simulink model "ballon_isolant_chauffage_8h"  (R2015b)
settings: Solver=ode23t  StartTime=0.0  StopTime=86400  RelTol=1e-3
undefined symbols (not defined in the file): sigbuilder_block
libraries: fl_lib x7, nesl_utility x4

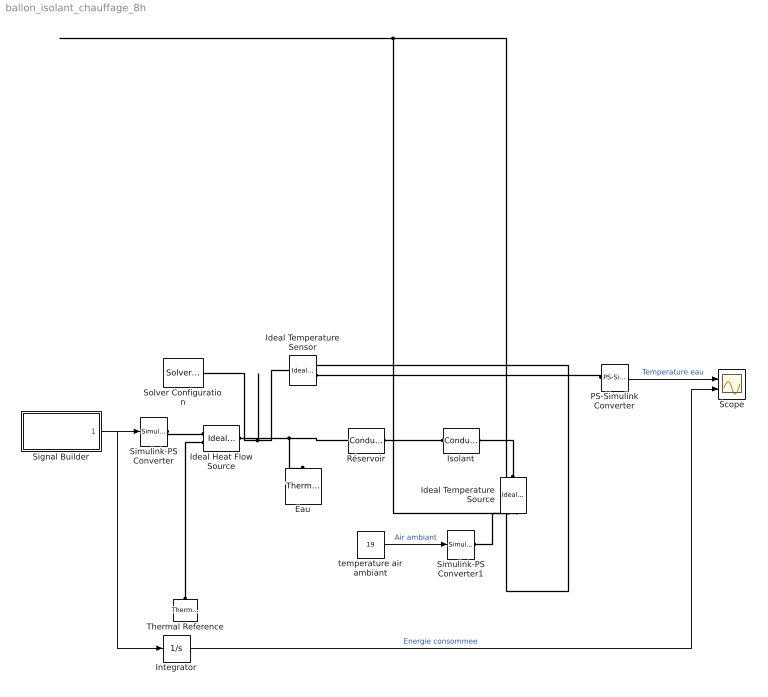
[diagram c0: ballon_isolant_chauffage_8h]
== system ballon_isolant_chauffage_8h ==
  Eau : fl_lib/Thermal/Thermal Elements/Thermal Mass  mass=300 kg  sp_heat=4185 J/kg/K  Q_specify=off  Q_priority=None  Q=0 J/s  T_specify=on  T_priority=High  T=15 C
  Ideal Temperature Source : fl_lib/Thermal/Thermal Sources/Ideal Temperature Source
  Ideal Heat Flow Source : fl_lib/Thermal/Thermal Sources/Ideal Heat Flow Source
  Ideal Temperature Sensor : fl_lib/Thermal/Thermal Sensors/Ideal Temperature Sensor
  Integrator : Integrator
  Isolant : fl_lib/Thermal/Thermal Elements/Conductive Heat Transfer  area=2.8 m^2  thickness=31 mm  th_cond=0.03 W/(m*K)  Q_specify=off  Q_priority=None  Q=0 J/s  T_specify=off  T_priority=None  T=0 K
  PS-Simulink Converter : nesl_utility/PS-Simulink Converter  PhysicalDomain=network_engine_domain  SubClassName=ps_output  LeftPortType=input  RightPortType=output  PseudoPeriodic=off  Frequencies=[]  Unit=C  AffineConversion=on
  Réservoir : fl_lib/Thermal/Thermal Elements/Conductive Heat Transfer  area=2.8 m^2  thickness=2 mm  th_cond=50 W/(m*K)  Q_specify=off  Q_priority=None  Q=0 J/s  T_specify=off  T_priority=None  T=0 K
  Scope : Scope  NumInputPorts=2
  Signal Builder : Subsystem  Tag=STV Subsys  LoadFcn=sigbuilder_block('load',[327 197.25 743.25 399.75 ]);  StartFcn=sigbuilder_block('start');  StopFcn=sigbuilder_block('stop');  ClipboardFcn=sigbuilder_block('clipboard');
  Simulink-PS Converter : nesl_utility/Simulink-PS Converter  PhysicalDomain=network_engine_domain  SubClassName=ps_input  LeftPortType=input  RightPortType=output  PseudoPeriodic=off  Frequencies=[]  NoiseDistribution=none  NoiseParameters=[]  Unit=W  AffineConversion=on  InputFiltering=off  SimscapeFilterOrder=1  InputFilterTimeConstant=.001  UdotUserProvided=0
  Simulink-PS Converter1 : nesl_utility/Simulink-PS Converter  PhysicalDomain=network_engine_domain  SubClassName=ps_input  LeftPortType=input  RightPortType=output  PseudoPeriodic=off  Frequencies=[]  NoiseDistribution=none  NoiseParameters=[]  Unit=C  AffineConversion=on  InputFiltering=off  SimscapeFilterOrder=1  InputFilterTimeConstant=.001  UdotUserProvided=1
  Solver Configuration : nesl_utility/Solver Configuration  PhysicalDomain=network_engine_domain  SubClassName=solver  LeftPortType=input  RightPortType=generic  Accelerate=off  Tones=[]  Harmonics=[]  SimulateNoise=off  Profile=off  UseLocalSampling=off  EnableSwitchedLinearOptims=on  FrequencyDomain=off  UseCCode=off  RelTol=0.001  AbsTol=1e-06  MinStep=1e-09  ToWorkspace=off  RevertToSquareIcSolve=off  NumHomotopyIterations=100  PhasorMode=off  PhasorModeNumHarmonics=1  DoDC=off  ResidualTolerance=1e-09  UseLocalSolver=off  LocalSolverChoice=NE_BACKWARD_EULER_ADVANCER  LocalSolverSampleTime=0.001  DoFixedCost=off  MaxNonlinIter=3  MaxModeIter=2  LinearAlgebra=Sparse  DelaysMemoryBudget=1024  AutomaticFiltering=on  FilteringTimeConstant=0.001
  Thermal Reference : fl_lib/Thermal/Thermal Elements/Thermal Reference
  temperature air ambiant : Constant  Value=19
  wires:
  Signal Builder/1(Signal 1) -> Simulink-PS Converter/1, Integrator/1
  PS-Simulink Converter/1 -> Scope/1  "Temperature eau"
  Integrator/1 -> Scope/2  "Energie consommee"
  temperature air ambiant/1 -> Simulink-PS Converter1/1  "Air ambiant"
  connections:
  Ideal Heat Flow Source/LConn1 -- Réservoir/LConn1 -- Eau/LConn1 -- Solver Configuration/RConn1 -- Ideal Temperature Sensor/LConn1
  Thermal Reference/LConn1 -- Ideal Temperature Sensor/RConn1 -- Ideal Temperature Source/RConn2 -- Ideal Heat Flow Source/RConn2
  Simulink-PS Converter/RConn1 -- Ideal Heat Flow Source/RConn1
  PS-Simulink Converter/LConn1 -- Ideal Temperature Sensor/RConn2
  Ideal Temperature Source/LConn1 -- Isolant/RConn1
  Simulink-PS Converter1/RConn1 -- Ideal Temperature Source/RConn1
  Isolant/LConn1 -- Réservoir/RConn1

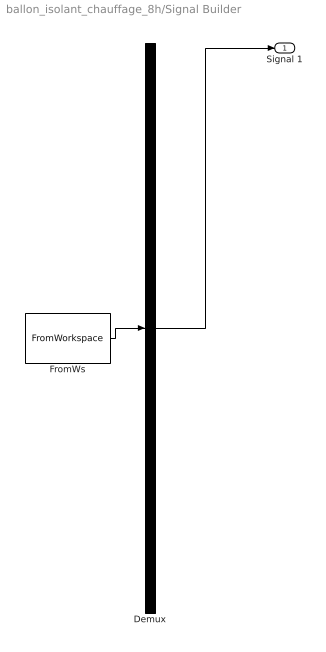
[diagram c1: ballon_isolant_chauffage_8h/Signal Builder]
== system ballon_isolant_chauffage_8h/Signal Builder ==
  Demux : Demux  Tag=STV Demux  Outputs=1
  FromWs : FromWorkspace  Tag=STV FromWs  VariableName=tuvar  SampleTime=0
  Signal 1 : Outport  Tag=STV Outport
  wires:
  Demux/1 -> Signal 1/1
  FromWs/1 -> Demux/1
